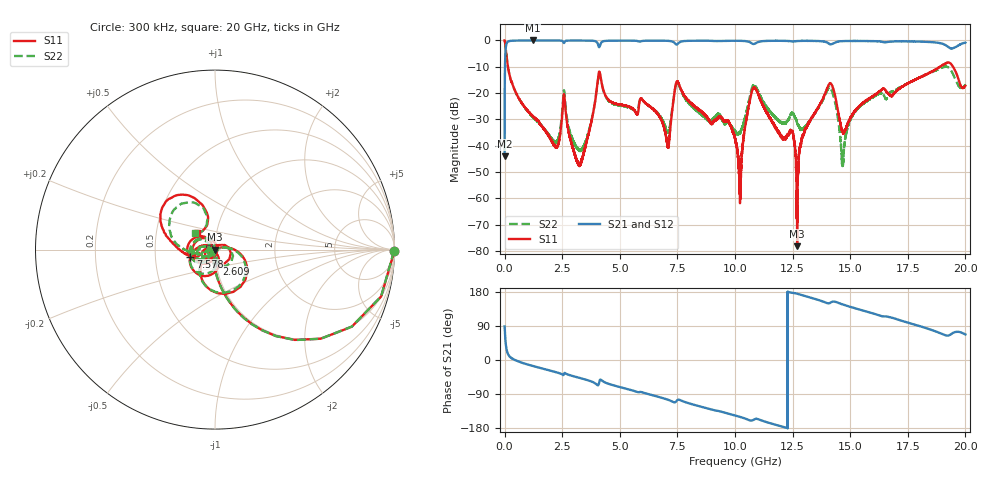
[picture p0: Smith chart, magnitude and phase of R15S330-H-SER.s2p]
!{R15S330}
!Johanson Technology Inc.
!www.johansontechnology.com
!Test Board Conditions:
!Substrate Type  RO4350B
!Substrate Thickness  20 mil
!Substrate Dk  3.66
!TL Type: GCPW
!TL Trace Width  34 mil
!TL Gap  10 mil
!Electrode orientation  Horizontal
!DUT TOPOLOGY	SERIES
!Mounting Pad LxW  26x52 mil
! Created Sat Feb  6 14:26:02 2021
# hz S ma R 50
! 2 Port Network Data from SP1.SP block
! freq  magS11  angS11  magS21  angS21  magS12  angS12  magS22  angS22
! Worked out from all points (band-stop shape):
!   20001 points, 300 kHz to 20 GHz, reference 50 ohm
!   highest |S21| = -0.01 dB at 1.218 GHz (marker M1); lowest = -44.0 dB at 300 kHz (marker M2)
!   |S21| within 3 dB of the highest: 47.82 MHz to 19.37 GHz (19.32 GHz wide, 199 % of centre); 19.45 GHz to end of sweep
!   lowest |S11| = -78.1 dB at 12.7 GHz (marker M3), VSWR 1.00, Z = 50 + j0.0116 ohm
!   |S11| at or under -10 dB: 143 MHz to 18.9 GHz (18.76 GHz wide, 197 % of centre); 19.46125 GHz to 19.46147 GHz (218.9 kHz wide, 0.00112 % of centre); 19.46 GHz to end of sweep
!   |S22| runs from -48.3 to 0.0 dB; largest |S21 - S12| = 0.015
!   S11 on the Smith chart (normalised r, x): 300 kHz: open; 2.609 GHz: 1.00, -0.16; 7.578 GHz: 0.76, -0.06; 20 GHz: 0.80, +0.15
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300000  0.9986 -0.5  0.006342 88.7  0.006271 89.4  0.9976 -0.4
1.373e8  0.328 -72.7  0.9428 17.1  0.9425 17.0  0.3288 -72.7
1.2183e9  0.03666 -111.6  0.999 -15.6  0.9976 -15.6  0.0357 -100.2
2.2413e9  0.00932 145.5  0.9968 -32.3  0.997 -32.3  0.01158 -35.9
2.6093e9  0.07745 -84.6  0.9386 -34.1  0.9381 -34.1  0.09077 -77.3
3.3343e9  0.005341 78.6  0.9957 -48.6  0.9952 -48.6  0.008423 -22.2
4.1153e9  0.256 -72.3  0.7523 -56.3  0.7517 -56.3  0.2479 -74.6
6.6673e9  0.03895 171.0  0.9901 -97.1  0.9903 -97.1  0.04044 -173.4
7.0913e9  0.00949 -129.8  0.9831 -104.9  0.9817 -104.8  0.01757 -128.1
7.5783e9  0.144 -163.5  0.914 -104.9  0.9147 -104.9  0.139 -166.2
1.00003e10  0.01356 128.6  0.9856 -146.3  0.9863 -146.3  0.01882 174.4
1.02373e10  0.002187 -106.7  0.9834 -150.5  0.9833 -150.5  0.0188 -150.5
1.08603e10  0.126 178.5  0.8684 -156.0  0.8686 -156.0  0.1377 176.9
1.24703e10  0.01905 -124.8  0.9599 177.4  0.9616 177.3  0.04209 -175.7
1.26983e10  0.0001243 69.1  0.9717 175.0  0.9729 174.9  0.02731 169.2
1.33343e10  0.03455 -103.4  0.9806 163.8  0.9814 163.6  0.03399 -127.1
1.41463e10  0.154 175.4  0.8415 151.4  0.845 151.3  0.127 164.9
1.46803e10  0.0182 163.3  0.973 146.5  0.9718 146.6  0.004238 -169.7
1.52233e10  0.04671 -133.7  0.9767 136.2  0.9777 136.6  0.04439 -133.9
1.66673e10  0.09575 -170.1  0.9428 113.6  0.9341 113.7  0.09148 -163.7
1.92363e10  0.3813 137.1  0.7643 64.5  0.7669 64.9  0.314 124.6
2e10  0.1377 138.8  0.9074 67.4  0.9042 67.2  0.1433 140.3
